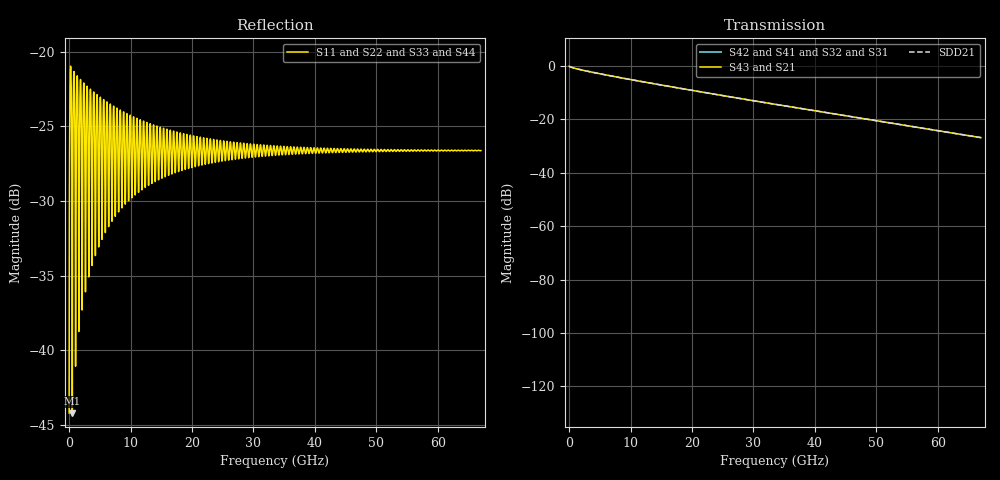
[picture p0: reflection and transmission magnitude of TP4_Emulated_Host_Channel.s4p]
! Created Tue Oct  9 17:58:46 2018
# hz S ma R 50
! 4 Port Network Data from SP1.SP block
! freq  magS11  angS11  magS12  angS12  magS13  angS13  magS14  angS14
!  magS21  angS21  magS22  angS22  magS23  angS23  magS24  angS24
!  magS31  angS31  magS32  angS32  magS33  angS33  magS34  angS34
!  magS41  angS41  magS42  angS42  magS43  angS43  magS44  angS44
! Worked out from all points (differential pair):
!   6700 points, 10 MHz to 67 GHz, reference 50 ohm
!   strongest paths, dB at 10 MHz, 16.76 GHz, 33.51 GHz, 50.26 GHz, 67 GHz:
!     S43: -0.1, -7.8, -14.3, -20.6, -26.8
!     S21: -0.1, -7.8, -14.3, -20.6, -26.8
!     S42: -180.0, -180.0, -180.0, -180.0, -180.0
!     S41: -180.0, -180.0, -180.0, -180.0, -180.0
!     S32: -180.0, -180.0, -180.0, -180.0, -180.0
!     S31: -180.0, -180.0, -180.0, -180.0, -180.0
!   taken as a pair (ports 3,1 in; 4,2 out), SDD21 dB: -0.1, -7.8, -14.3, -20.6, -26.8
!   lowest |S11| = -44.2 dB at 530 MHz (marker M1), VSWR 1.01, Z = 50.6 + j0.207 ohm
!   |S11| at or under -10 dB: start of sweep to end of sweep
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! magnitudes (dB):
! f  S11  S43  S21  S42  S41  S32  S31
! 10 MHz  -44.2  -0.1  -0.1  -180.0  -180.0  -180.0  -180.0
! 530 MHz  -44.2  -0.6  -0.6  -180.0  -180.0  -180.0  -180.0
! 790 MHz  -21.3  -0.8  -0.8  -180.0  -180.0  -180.0  -180.0
! 1.05 GHz  -40.1  -0.9  -0.9  -180.0  -180.0  -180.0  -180.0
! 1.33 GHz  -21.6  -1.1  -1.1  -180.0  -180.0  -180.0  -180.0
! 1.59 GHz  -38.7  -1.2  -1.2  -180.0  -180.0  -180.0  -180.0
! 67 GHz  -26.6  -26.8  -26.8  -180.0  -180.0  -180.0  -180.0
